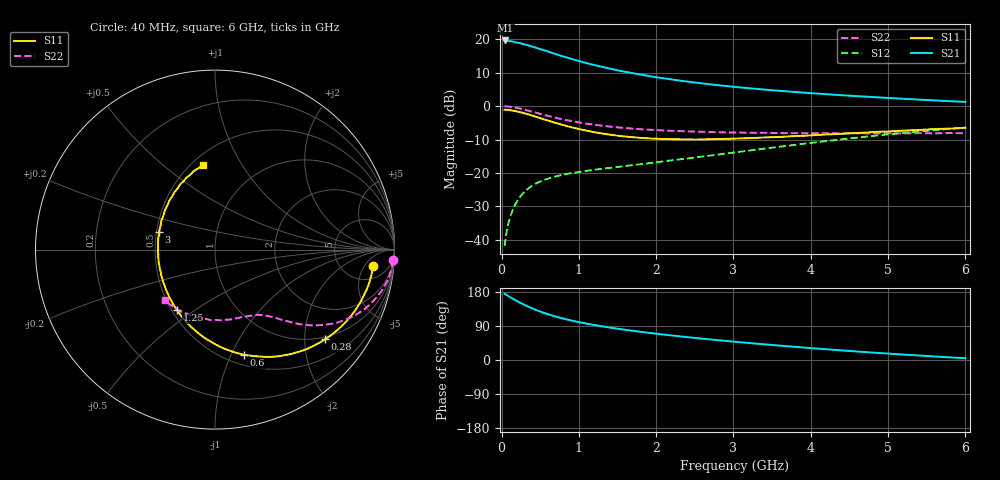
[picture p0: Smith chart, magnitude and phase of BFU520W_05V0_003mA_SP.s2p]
! Filename:  P:\Prog\Test\Noise\ATS_data\Testdata_Net\Run2\BFU520W_APM2013_06_A05_05p0V_003mA_SP_CM01_D.s2p
! Date/Time: Tue 26/Mar/2013 18:01:40
! BFU520W_APM2013_06_A05_05p0V_1to20mA_SP_CM01_Bias3_R.s2p
! MDIF S-parameter v. bias file
! BFU520W_APM2013_06_A05_05p0V_1to20mA_SP_CM01
! Date/time Thu Mar 21 14:22:37 2013
! VAR V_out= 5.0010
! VAR I_out= 3.0050
! VAR V_in= 0.8186
! VAR I_in= 0.0334
! Device data file deembeded for feedlines and parallel
! Original file: \Run2\BFU520W_APM2013_06_A05_05p0V_003mA_SP_CM01_R.s2p
! Feed-files: PR019V01_070313_Feed1.s2p, PR019V01_070313_Feed2.s2p
! Parallel-file: PR019V01_070313_Par.s2p
# MHz S MA R 50
!  Freq-MHz  S11-mag  S11-arg  S21-mag  S21-arg  S12-mag  S12-arg  S22-mag  S22-arg
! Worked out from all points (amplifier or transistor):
!   98 points, 40 MHz to 6 GHz, reference 50 ohm
!   highest |S21| = 19.7 dB at 50 MHz (marker M1)
!   |S21| within 3 dB of that: start of sweep to 558.5 MHz
!   unconditionally stable (mu >= 1): 2.117 GHz to 3.292 GHz
!   at 300 MHz: K = 0.23, MSG = 22.0 dB, |S12| = -25.6 dB
!   at 1.6 GHz: K = 0.90, MSG = 14.1 dB, |S12| = -17.9 dB
!   at 6 GHz: K = 0.84, MSG = 3.9 dB, |S12| = -6.4 dB
!   S11 on the Smith chart (normalised r, x): 40 MHz: 10, -8; 280 MHz: 0.94, -2.51; 600 MHz: 0.60, -1.12; 1.25 GHz: 0.53, -0.43; 3 GHz: 0.52, +0.11; 6 GHz: 0.57, +0.69
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40  0.8857 -5.9  9.613 174.8  0.00802 85.8  0.995 -3.4
50  0.8852 -7.4  9.624 173.4  0.009968 85.6  0.9936 -4.2
120  0.8668 -17.6  9.393 164.7  0.02344 79.8  0.9757 -10.1
160  0.852 -23.2  9.174 160.1  0.03078 76.6  0.9602 -13.3
240  0.8123 -34.1  8.782 151.2  0.04388 71.0  0.9191 -19.1
280  0.7918 -39.1  8.487 147.1  0.04981 68.5  0.8967 -21.7
340  0.7566 -46.8  8.172 141.3  0.05767 65.1  0.8597 -25.3
420  0.7085 -56.0  7.655 134.2  0.06688 61.3  0.8124 -29.3
500  0.6619 -64.6  7.146 127.9  0.07451 58.1  0.7671 -32.7
600  0.6087 -74.5  6.581 120.8  0.08232 55.2  0.7146 -36.1
700  0.5607 -83.3  6.029 114.7  0.08877 53.0  0.67 -39.0
800  0.5196 -91.3  5.539 109.3  0.0943 51.5  0.6319 -41.2
900  0.4852 -99.0  5.117 104.4  0.09923 50.5  0.5996 -42.9
1050  0.4422 -109.4  4.574 98.0  0.1055 49.8  0.558 -45.3
1250  0.3982 -122.0  3.997 90.5  0.1134 49.6  0.518 -47.8
1600  0.3515 -141.4  3.27 79.7  0.1269 50.8  0.4705 -51.7
2050  0.3238 -162.4  2.659 68.2  0.1466 53.3  0.4353 -56.7
3000  0.3266 162.5  1.952 48.5  0.2018 56.9  0.403 -70.2
3100  0.3293 159.4  1.901 46.7  0.2087 57.0  0.4022 -71.7
4100  0.3717 133.7  1.539 29.9  0.2908 55.3  0.3914 -90.4
5200  0.4309 111.8  1.289 14.3  0.3974 48.0  0.3898 -114.6
6000  0.4753 98.4  1.157 4.7  0.4765 40.5  0.3937 -134.5
